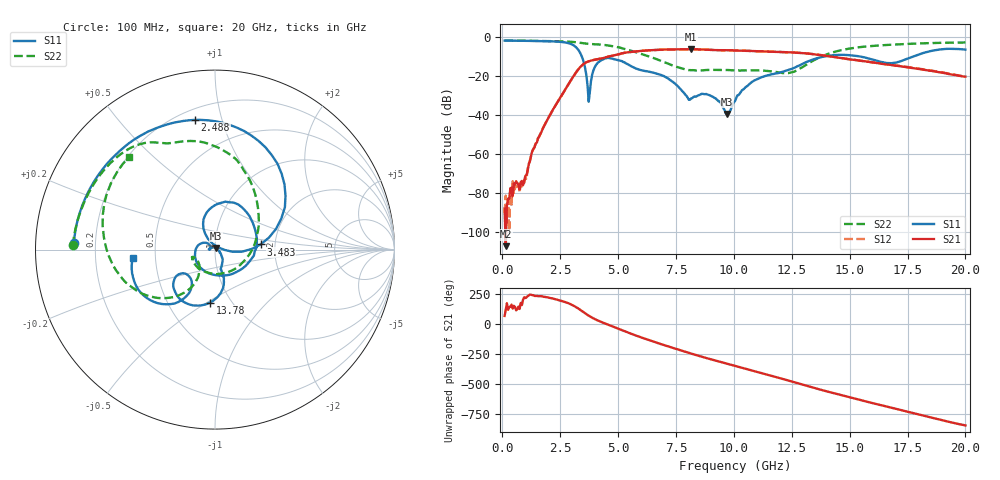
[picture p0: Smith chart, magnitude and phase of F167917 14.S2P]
!  2-Port S-parameters saved by WinCal
! VAR MeasName=S-Parameters (CALIBRATED_DATA) read from VNA (N5242A)
! VAR MeasDate=2016-11-22 9:00:22
! VAR NAME=F167917 14
! VAR FILENAME=F167917 14.S2P
! VAR DATE=2016-11-22 9:00:22
! VAR PHYS_PORTS=1,2
# Hz S DB R 50
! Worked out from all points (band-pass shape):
!   401 points, 100 MHz to 20 GHz, reference 50 ohm
!   highest |S21| = -6.51 dB at 8.159 GHz (marker M1); lowest = -107.5 dB at 149.8 MHz (marker M2)
!   |S21| within 3 dB of the highest: 4.889 GHz to 13.72 GHz (8.834 GHz wide, 94.9 % of centre)
!   lowest |S11| = -39.7 dB at 9.702 GHz (marker M3), VSWR 1.02, Z = 50.3 + j0.974 ohm
!   |S11| at or under -10 dB: 3.425 GHz to 14.02 GHz (10.59 GHz wide, 121 % of centre); 15.32 GHz to 17.79 GHz (2.476 GHz wide, 15 % of centre)
!   |S22| runs from -18.8 to -2.0 dB; largest |S21 - S12| = 0.0042
!   S11 on the Smith chart (normalised r, x): 100 MHz: 0.12, +0.02; 2.488 GHz: 0.26, +0.82; 3.483 GHz: 1.68, +0.10; 13.78 GHz: 0.80, -0.52; 20 GHz: 0.37, -0.05
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1e8  -2.09 177.3  -88.27 66.3  -90.27 177.9  -2.03 178.3
1.4975e8  -2.09 176.0  -107.46 121.4  -81.58 175.1  -2.03 177.5
9.4575e8  -2.21 154.7  -73.92 -138.6  -75.03 -165.2  -2.16 165.0
1.34375e9  -2.28 143.3  -57.66 -121.5  -57.74 -123.3  -2.23 158.8
2.488e9  -2.72 98.8  -31.70 -164.7  -31.71 -165.2  -2.45 138.8
3.43325e9  -10.21 12.6  -14.89 107.9  -14.89 107.9  -3.40 118.1
3.483e9  -11.84 6.5  -14.39 101.3  -14.36 101.2  -3.49 117.3
3.73175e9  -33.44 37.6  -12.73 68.9  -12.71 68.8  -3.80 113.4
4.03025e9  -14.89 110.8  -11.82 37.4  -11.80 37.1  -4.00 107.6
4.52775e9  -11.00 68.5  -10.46 -2.9  -10.47 -3.3  -4.52 94.4
5.72175e9  -16.14 -66.9  -7.71 -92.4  -7.69 -92.4  -7.87 58.3
6.7665e9  -19.31 -179.1  -6.80 -161.6  -6.80 -161.8  -12.09 19.2
8.1595e9  -31.71 171.3  -6.51 114.7  -6.51 114.6  -17.29 -81.6
8.90575e9  -29.90 170.1  -6.82 72.4  -6.82 72.3  -17.13 -128.0
9.70175e9  -39.74 69.8  -7.03 30.4  -7.04 30.5  -17.15 -152.3
1.005e10  -33.08 -19.3  -7.16 11.8  -7.17 11.9  -17.39 -157.3
1.179125e10  -18.98 -73.5  -7.86 -78.9  -7.83 -78.8  -18.13 -160.0
1.338325e10  -11.94 -84.4  -8.98 -165.6  -8.94 -165.1  -12.64 -121.5
1.378125e10  -10.56 -95.4  -9.58 173.1  -9.53 173.5  -10.26 -126.7
1.67165e10  -13.68 -136.0  -14.45 29.8  -14.42 30.1  -4.27 177.3
1.85075e10  -7.44 -134.5  -17.59 -55.1  -17.42 -55.6  -3.37 152.3
2e10  -6.70 -173.9  -20.58 -121.6  -20.46 -122.2  -3.06 132.8
